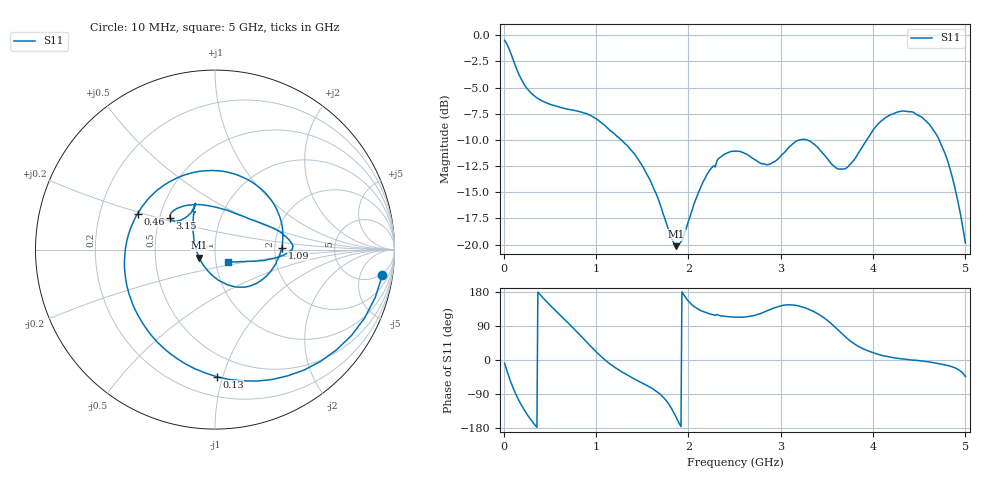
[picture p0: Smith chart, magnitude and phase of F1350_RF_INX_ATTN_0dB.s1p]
! S-parameters for RF_INX input IDT F1350 DPD Demodulator
! Date Measured:  2015-11-25  RGG
!  Port 1 = Pin 35 = RF_INX
! STATE: RF_INX selected, 0 dB attenuation (Gain = Gmax - 0 dB)
! RF Frequency:  10 MHz to 5000 MHz
! RF_INY, IF_I+, IF_I-, IF_Q+, and IF_Q- terminated
! 2300 MHz, 0 dBm signal applied to LO_IN
! Vcc = +5.00 Volts  Icc = approx 275 mA.
! NOTES:  The device was measured on a custom printed circuit evaluation board with individual 50 ohm
!  microstrip lines to the RF and LO pins. The 50 ohm microstrip lines were de-embedded using reference
!  plane extensions
! Instrument Manufacturer:  Agilent Technologies
! Instrument Model:  E5071C
! Instrument Serial Number:  MY46419053
! Instrument Firmware Rev:  A.11.31
! Frequency Re{S11} Im{S11}
# HZ  S  RI R 50.00
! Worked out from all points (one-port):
!   500 points, 10 MHz to 5 GHz, reference 50 ohm
!   lowest |S11| = -20.2 dB at 1.87 GHz (marker M1), VSWR 1.22, Z = 41.8 - j3.86 ohm
!   |S11| at or under -10 dB: 1.272 GHz to 3.208 GHz (1.936 GHz wide, 86.4 % of centre); 3.282 GHz to 3.932 GHz (650 MHz wide, 18 % of centre); 4.716 GHz to end of sweep
!   S11 on the Smith chart (normalised r, x): 10 MHz: 4, -11; 130 MHz: 0.34, -0.96; 460 MHz: 0.37, +0.19; 1.09 GHz: 2.18, +0.06; 3.15 GHz: 0.57, +0.22; 5 GHz: 1.15, -0.16
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1e7  0.9327 -0.1425
7e7  0.4971 -0.6708
1.3e8  0.00953 -0.7082
1.9e8  -0.2916 -0.5445
2.6e8  -0.4564 -0.3102
3.5e8  -0.5037 -0.0454
4.6e8  -0.4317 0.2002
6.4e8  -0.1648 0.4176
8.3e8  0.1822 0.39
9.6e8  0.3473 0.2162
1.09e9  0.3721 0.0112
1.26e9  0.2817 -0.1515
1.55e9  0.0844 -0.1999
1.87e9  -0.087 -0.0457
1.89e9  -0.0948 -0.0303
2.21e9  -0.1197 0.1832
2.51e9  -0.109 0.2572
2.87e9  -0.1595 0.181
3.13e9  -0.2488 0.1726
3.15e9  -0.2504 0.1785
3.35e9  -0.1903 0.2371
3.61e9  0.0326 0.2287
3.76e9  0.1596 0.1842
4.08e9  0.3764 0.0881
4.38e9  0.4315 0.00718
4.73e9  0.3013 -0.0539
4.86e9  0.1978 -0.0651
5e9  0.0731 -0.0705
